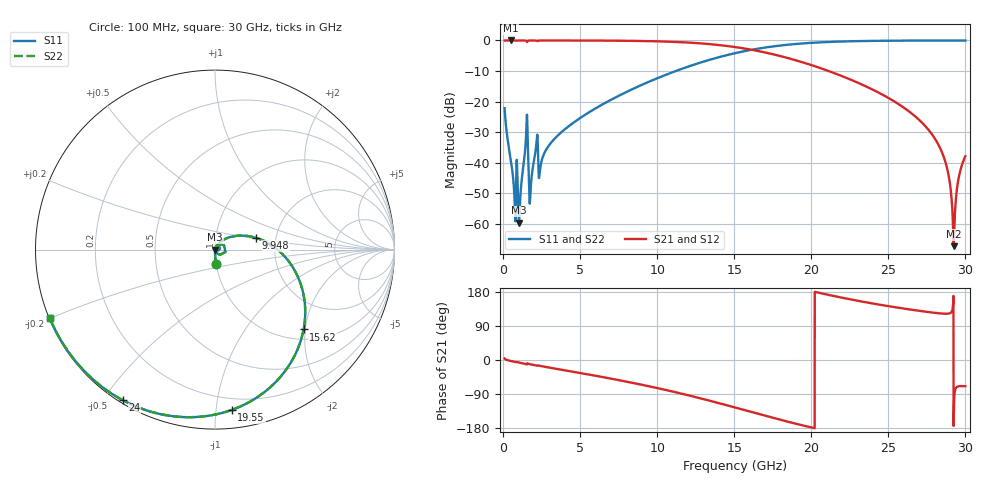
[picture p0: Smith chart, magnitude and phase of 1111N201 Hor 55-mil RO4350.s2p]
# GHz S MA R 50
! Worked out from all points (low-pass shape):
!   3201 points, 100 MHz to 30 GHz, reference 50 ohm
!   highest |S21| = 0.00 dB at 492.4 MHz (marker M1); lowest = -67.3 dB at 29.24 GHz (marker M2)
!   |S21| within 3 dB of the highest: start of sweep to 16.08 GHz
!   lowest |S11| = -59.6 dB at 1.034 GHz (marker M3), VSWR 1.00, Z = 50.1 + j0.0111 ohm
!   |S11| at or under -10 dB: start of sweep to 11.21 GHz
!   |S22| runs from -59.6 to 0.0 dB; largest |S21 - S12| = 0
!   S11 on the Smith chart (normalised r, x): 100 MHz: 1.00, -0.16; 9.948 GHz: 1.57, +0.22; 15.62 GHz: 1.23, -1.96; 19.55 GHz: 0.12, -1.10; 24 GHz: 0.01, -0.56; 30 GHz: 0.00, -0.20
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0.1  0.07799 -86.0  0.9967 3.8  0.9967 3.8  0.07799 -86.0
0.4924375  0.0115 -90.5  0.9995 -2.5  0.9995 -2.5  0.0115 -90.5
0.6886562  0.004463 -87.3  0.9994 -4.1  0.9994 -4.1  0.004463 -87.3
1.034375  0.001053 6.0  0.9989 -6.6  0.9989 -6.6  0.001053 6.0
1.482875  0.02472 64.6  0.9933 -10.8  0.9933 -10.8  0.02472 64.6
1.800563  0.004098 56.1  0.9982 -11.6  0.9982 -11.6  0.004098 56.1
2.11825  0.01643 64.7  0.9965 -14.3  0.9965 -14.3  0.01643 64.7
2.435938  0.008914 61.9  0.9978 -15.9  0.9978 -15.9  0.008914 61.9
5.089563  0.05583 54.0  0.9967 -34.9  0.9967 -34.9  0.05583 54.0
9.948313  0.2378 16.0  0.9682 -73.5  0.9682 -73.5  0.2378 16.0
10.06978  0.2447 14.9  0.9664 -74.6  0.9664 -74.6  0.2447 14.9
15.05  0.6188 -35.7  0.7799 -125.3  0.7799 -125.3  0.6188 -35.7
15.61997  0.6645 -42.0  0.7412 -131.7  0.7412 -131.7  0.6645 -42.0
19.55369  0.898 -84.0  0.4301 -173.7  0.4301 -173.7  0.898 -84.0
20.03956  0.9148 -88.7  0.3931 -178.3  0.3931 -178.3  0.9148 -88.7
24.00131  0.9839 -121.4  0.1564 149.0  0.1564 149.0  0.9839 -121.4
25.01978  0.9898 -128.5  0.1143 142.0  0.1143 142.0  0.9898 -128.5
28.19666  0.9962 -147.9  0.02093 123.6  0.02093 123.6  0.9962 -147.9
28.83203  0.9964 -151.4  0.007753 122.1  0.007753 122.1  0.9964 -151.4
29.24316  0.9965 -153.6  0.0004338 -152.4  0.0004338 -152.4  0.9965 -153.6
29.58888  0.9964 -155.5  0.006095 -69.2  0.006095 -69.2  0.9964 -155.5
30  0.9964 -157.6  0.01281 -69.2  0.01281 -69.2  0.9964 -157.6
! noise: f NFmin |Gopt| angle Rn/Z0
0.1  0.0006565  0.7312  0.8565  0.0004867
3.417  0.008407  0.4182  20.86  0.002295
6.743  0.01418  0.3618  38.25  0.003191
10.06  0.02124  0.3794  52.9  0.004575
13.39  0.03128  0.4461  66.78  0.006972
16.7  0.04802  0.5583  82.35  0.01173
20.03  0.08152  0.6998  100.7  0.02263
23.35  0.1651  0.8368  120.4  0.05414
26.67  0.5095  0.9432  139.7  0.2398
30  2.353  0.9868  157.5  1.632
